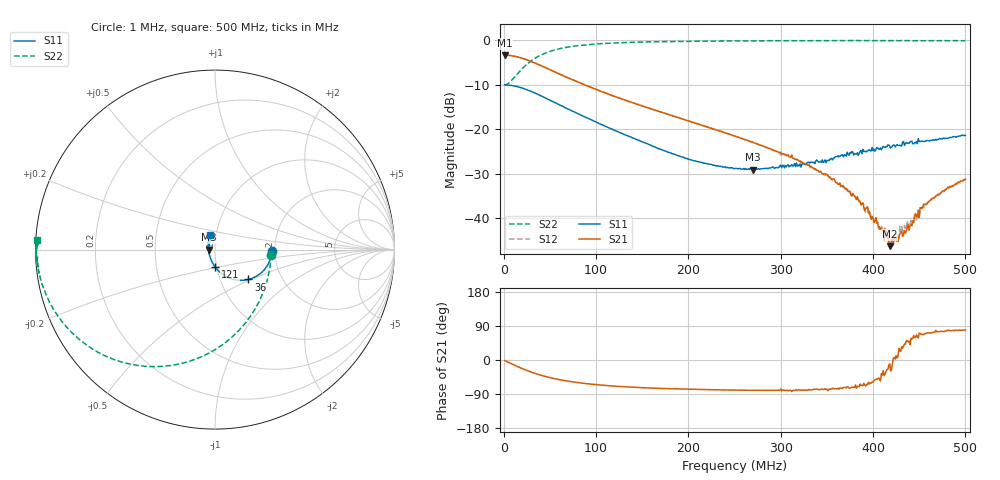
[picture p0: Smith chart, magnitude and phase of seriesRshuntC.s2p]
# Hz S RI R 50.0
! written by SimSmith version 18.3b
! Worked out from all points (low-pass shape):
!   500 points, 1 MHz to 500 MHz, reference 50 ohm
!   highest |S21| = -3.31 dB at 1 MHz (marker M1); lowest = -46.3 dB at 418 MHz (marker M2)
!   |S21| within 3 dB of the highest: start of sweep to 47.03 MHz
!   lowest |S11| = -29.1 dB at 270 MHz (marker M3), VSWR 1.07, Z = 46.6 - j0.0947 ohm
!   |S11| at or under -10 dB: 1.761 MHz to end of sweep
!   |S22| runs from -10.0 to 0.0 dB; largest |S21 - S12| = 0.0043
!   S11 on the Smith chart (normalised r, x): 1 MHz: 1.93, -0.03; 36 MHz: 1.36, -0.48; 121 MHz: 0.98, -0.19; 500 MHz: 0.93, +0.15
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1000000  0.3167 -0.00752  0.6831 -0.0147  0.6833 -0.0148  0.3134 -0.0277
1e7  0.3015 -0.0699  0.6551 -0.1364  0.6552 -0.1364  0.2586 -0.2611
2e7  0.2634 -0.1239  0.5816 -0.2425  0.5821 -0.2429  0.1191 -0.4649
3.6e7  0.1862 -0.1662  0.4347 -0.3269  0.4351 -0.3283  -0.1622 -0.6281
6e7  0.0946 -0.1636  0.2607 -0.3295  0.26 -0.3314  -0.4977 -0.632
8.5e7  0.0401 -0.136  0.1572 -0.2836  0.1556 -0.2857  -0.6968 -0.5433
1.21e8  0.000527 -0.0962  0.0829 -0.2171  0.0808 -0.2187  -0.8411 -0.415
1.68e8  -0.0215 -0.0563  0.0416 -0.1533  0.0389 -0.1542  -0.9231 -0.2894
2.04e8  -0.0296 -0.0335  0.0263 -0.1176  0.0238 -0.1182  -0.9531 -0.2208
2.51e8  -0.0351 -0.00924  0.0152 -0.0819  0.0132 -0.0822  -0.9756 -0.1502
2.7e8  -0.035 -0.00101  0.0126 -0.07  0.0107 -0.0701  -0.9818 -0.127
3.34e8  -0.0348 0.0249  0.00728 -0.0362  0.00608 -0.0366  -0.9933 -0.0627
3.83e8  -0.0338 0.0424  0.00611 -0.0163  0.00619 -0.0159  -0.9965 -0.021
4.15e8  -0.0326 0.0541  0.00603 -0.0029  0.00664 -0.00279  -0.9938 0.007
4.17e8  -0.0363 0.0553  0.00489 -0.00126  0.00507 -0.00167  -0.9953 0.00604
4.18e8  -0.0335 0.0561  0.00474 -0.000837  0.00526 -0.000837  -0.9946 0.00682
4.26e8  -0.0306 0.0597  0.0055 0.000528  0.00654 0.00077  -0.9981 0.0139
4.3e8  -0.0297 0.0577  0.00643 0.0027  0.00651 0.00254  -0.9944 0.0174
4.34e8  -0.0317 0.0578  0.00532 0.00483  0.00656 0.00497  -0.9943 0.0154
4.53e8  -0.0288 0.0673  0.00499 0.0118  0.00593 0.0118  -0.9944 0.0281
4.77e8  -0.0296 0.0739  0.00529 0.0194  0.00673 0.0186  -0.9939 0.04
5e8  -0.0284 0.0801  0.00526 0.0269  0.0072 0.0258  -0.9922 0.054
